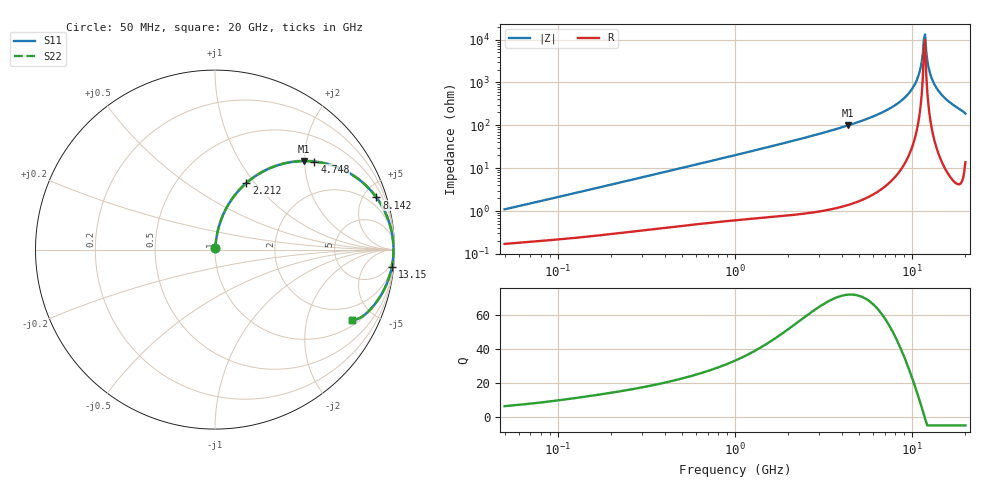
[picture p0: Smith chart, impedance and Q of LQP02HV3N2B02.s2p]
!Murata Part Number: LQP02HV3N2B02
!These Parameters are Measured in Series Mode Connection
!  o--[Z]--o
!Port1  Port2
!  o-------o
!Freq. Start=50[MHz] Stop=20[GHz], 401[Steps]
# Hz S RI R 50
!Freq.(Hz) S11(Real) S11(Imag) S21(Real) S21(Imag) S12(Real) S12(Imag) S22(Real) S22(Imag)
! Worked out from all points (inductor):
!   401 points, 50 MHz to 20 GHz, reference 50 ohm
!   read as one part in series: L = 3.41 nH near 51.52 MHz
!   highest Q = 71.8 at 4.34 GHz (marker M1), where L = 3.63 nH
!   self-resonance near 11.66 GHz
!   S11 on the Smith chart (normalised r, x): 50 MHz: 1.00, +0.02; 2.212 GHz: 1.02, +0.91; 4.748 GHz: 1.03, +2.23; 8.142 GHz: 1.13, +6.14; 13.15 GHz: 2, -21; 20 GHz: 1.28, -3.73
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5e7  0.00182 0.0108  0.9982 -0.0108  0.9982 -0.0108  0.00182 0.0108
1.364002e8  0.00325 0.0283  0.9968 -0.0283  0.9968 -0.0283  0.00325 0.0283
3.721004e8  0.0095 0.0746  0.9905 -0.0746  0.9905 -0.0746  0.0095 0.0746
1e9  0.044 0.1905  0.956 -0.1905  0.956 -0.1905  0.044 0.1905
2.211938e9  0.1746 0.3706  0.8254 -0.3706  0.8254 -0.3706  0.1746 0.3706
2.728004e9  0.2479 0.4238  0.7521 -0.4238  0.7521 -0.4238  0.2479 0.4238
4.34015e9  0.4948 0.4931  0.5052 -0.4931  0.5052 -0.4931  0.4948 0.4931
4.748272e9  0.5543 0.4901  0.4457 -0.4901  0.4457 -0.4901  0.5543 0.4901
7.442007e9  0.8514 0.3464  0.1486 -0.3464  0.1486 -0.3464  0.8514 0.3464
8.141811e9  0.8989 0.2907  0.1011 -0.2907  0.1011 -0.2907  0.8989 0.2907
9.316812e9  0.9544 0.1934  0.0456 -0.1934  0.0456 -0.1934  0.9544 0.1934
1.034674e10  0.9818 0.1092  0.0182 -0.1092  0.0182 -0.1092  0.9818 0.1092
1.098561e10  0.9907 0.0589  0.00934 -0.0589  0.00934 -0.0589  0.9907 0.0589
1.115139e10  0.9921 0.0462  0.00795 -0.0462  0.00795 -0.0462  0.9921 0.0462
1.149051e10  0.9939 0.0206  0.00615 -0.0206  0.00615 -0.0206  0.9939 0.0206
1.166392e10  0.9943 0.0078  0.00574 -0.0078  0.00574 -0.0078  0.9943 0.0078
1.201863e10  0.9941 -0.0178  0.00593 0.0178  0.00593 0.0178  0.9941 -0.0178
1.257102e10  0.9913 -0.0563  0.00871 0.0563  0.00871 0.0563  0.9913 -0.0563
1.314879e10  0.9855 -0.0943  0.0145 0.0943  0.0145 0.0943  0.9855 -0.0943
1.396067e10  0.9733 -0.1442  0.0267 0.1442  0.0267 0.1442  0.9733 -0.1442
1.527346e10  0.9454 -0.2158  0.0546 0.2158  0.0546 0.2158  0.9454 -0.2158
2e10  0.7615 -0.3906  0.2385 0.3906  0.2385 0.3906  0.7615 -0.3906
